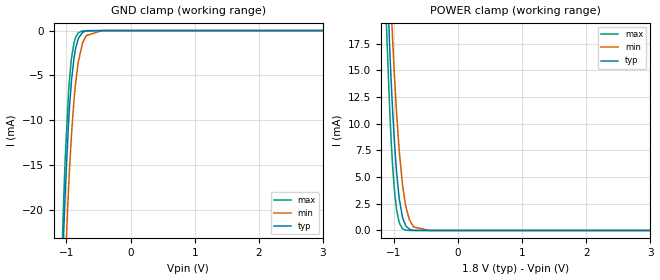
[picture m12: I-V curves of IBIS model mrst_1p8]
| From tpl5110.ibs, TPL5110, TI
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|   Model
[Model]   mrst_1p8
Model_type   Input
Vinl = 0.54
Vinh = 1.26
|   typ   min   max
C_comp   0.404pF   0.345pF   0.463pF
[Voltage Range]   1.8   1.71   1.89
[Temperature Range]   25   105   -40
[Power Clamp Reference]   1.8   1.71   1.89
[GND Clamp Reference]   0   0   0
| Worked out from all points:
|   GND clamp passes 1 mA (typ) near -0.82 V on its own axis
|   POWER clamp passes 1 mA (typ) near -0.85 V on its own axis
[GND Clamp]
|   Voltage   I(typ)   I(min)   I(max)
-1.8V     -269.1mA   -256mA     -288mA
-1.093V   -33.93mA   -41.65mA   -30.89mA
-1.044V   -23.12mA   -31.24mA   -19.4mA
-1.039V   -22.04mA   -30.17mA   -18.28mA
-1.017V   -17.99mA   -26.05mA   -14.18mA
-952.2mV  -8.645mA   -15.64mA   -5.507mA
-919.8mV  -5.559mA   -11.6mA    -3.068mA
-882mV    -3.111mA   -7.876mA   -1.404mA
-811.8mV  -863uA     -3.424mA   -243.6uA
-693mV    -45.4uA    -573.6uA   -3.817uA
-444.6mV  -3.111nA   -1.673uA   0A
3.6V      0A         0A         0A
[POWER Clamp]
|   Voltage   I(typ)   I(min)   I(max)
-1.8V     177.4mA    171.8mA    183.6mA
-1.114V   24.86mA    31.59mA    18.98mA
-1.066V   17.28mA    24.18mA    11.44mA
-1.033V   12.93mA    19.7mA     7.474mA
-1.022V   11.62mA    18.31mA    6.367mA
-990mV    8.172mA    14.42mA    3.705mA
-919.8mV  3.167mA    7.757mA    813.9uA
-860.4mV  1.145mA    4.066mA    142.7uA
-811.8mV  419.7uA    2.196mA    23.16uA
-693mV    15.38uA    335.2uA    102nA
-444.6mV  0A         725.3nA    0A
3.6V      0A         0A         0A
